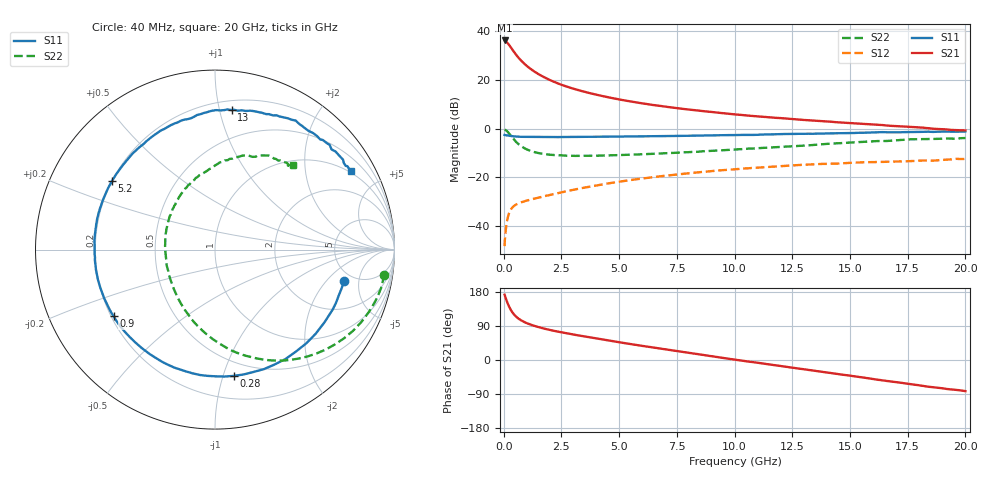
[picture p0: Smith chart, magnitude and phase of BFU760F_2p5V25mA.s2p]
! Filename:  P:\Prog\Test\Noise\ATS_data\Testdata_Net\Split files Spar\BFU760F_2W_C1_Bias6_2.5V_5mA_30mA_D.s2p
! Date/Time: Mon 06/Feb/2012 15:08:25
! BFU760_2W_C1_Bias6_2.5V_5mA_30mA_R.s2p
! MDIF S-parameter v. bias file
! BFU760_2W_C1_2.5V_5mA_30mA
! Date/time Fri Mar 18 11:16:19 2011
! VAR V_out= 2.5000
! VAR I_out= 24.9500
! VAR V_in= 0.7862
! VAR I_in= 0.0794
! Device data file deembeded for feedlines and parallel
! Original file: \Split files Spar\BFU760_2W_C1_Bias6_2.5V_5mA_30mA_R.s2p
! Feed-files: PR003V01_101208_Feed1.s2p, PR003V01_101208_Feed2.s2p
! Parallel-file: PR003V01_101208_Par.s2p
# MHz S MA R 50
!  Freq-MHz  S11-mag  S11-arg  S21-mag  S21-arg  S12-mag  S12-arg  S22-mag  S22-arg
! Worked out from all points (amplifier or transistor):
!   167 points, 40 MHz to 20 GHz, reference 50 ohm
!   highest |S21| = 36.2 dB at 40 MHz (marker M1)
!   |S21| within 3 dB of that: start of sweep to 320.2 MHz
!   unconditionally stable (mu >= 1): 3.954 GHz to 13.79 GHz
!   at 550 MHz: K = 0.30, MSG = 30.6 dB, |S12| = -31.1 dB
!   at 4.2 GHz: K = 1.01, MAG = 17.6 dB, |S12| = -23.0 dB
!   at 20 GHz: K = 0.90, MSG = 5.9 dB, |S12| = -12.5 dB
!   S11 on the Smith chart (normalised r, x): 40 MHz: 4.14, -3.20; 280 MHz: 0.38, -1.08; 900 MHz: 0.21, -0.29; 5.2 GHz: 0.20, +0.29; 13 GHz: 0.27, +1.09; 20 GHz: 0.94, +3.49
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40  0.7404 -13.6  64.42 172.3  0.003881 72.4  0.9544 -8.4
50  0.7375 -17.4  64.16 169.9  0.005298 72.3  0.9508 -10.9
90  0.7326 -30.4  62.42 162.8  0.008411 71.5  0.9322 -19.9
160  0.7253 -51.7  57.53 151.3  0.01392 64.5  0.8721 -34.5
220  0.7195 -67.8  53.12 142.7  0.01772 58.7  0.8092 -45.6
280  0.7114 -81.6  48.5 135.3  0.02072 53.8  0.7463 -55.4
400  0.6977 -103.4  40.24 123.8  0.02483 46.6  0.6325 -71.3
480  0.6921 -114.2  35.62 118.0  0.0267 43.3  0.5734 -80.1
550  0.6864 -122.0  32.3 113.8  0.02792 41.4  0.5272 -86.8
700  0.6804 -134.6  26.57 106.8  0.03014 38.8  0.4578 -98.6
900  0.6763 -146.6  21.32 99.9  0.03234 37.5  0.3961 -111.2
1300  0.6735 -161.6  15.15 90.6  0.03637 37.6  0.333 -129.8
1800  0.6718 -173.4  11.04 82.2  0.0415 39.1  0.2992 -146.0
2450  0.6729 176.3  8.11 73.7  0.04867 40.9  0.2833 -160.8
3400  0.6784 164.5  5.87 63.1  0.06045 41.0  0.2773 -176.4
5200  0.6899 146.3  3.819 44.9  0.08424 36.7  0.2893 161.5
6800  0.7025 132.2  2.91 29.9  0.1055 29.9  0.3095 145.5
10200  0.7429 104.8  1.927 -0.7  0.149 11.2  0.3785 115.9
13000  0.7829 83.2  1.508 -24.5  0.1815 -6.4  0.4489 94.2
13400  0.7842 80.7  1.463 -27.8  0.1855 -9.5  0.4616 91.3
16800  0.8428 54.8  1.14 -56.9  0.2105 -31.2  0.5658 66.2
20000  0.8742 30.1  0.9182 -82.2  0.2384 -52.9  0.6417 47.4
